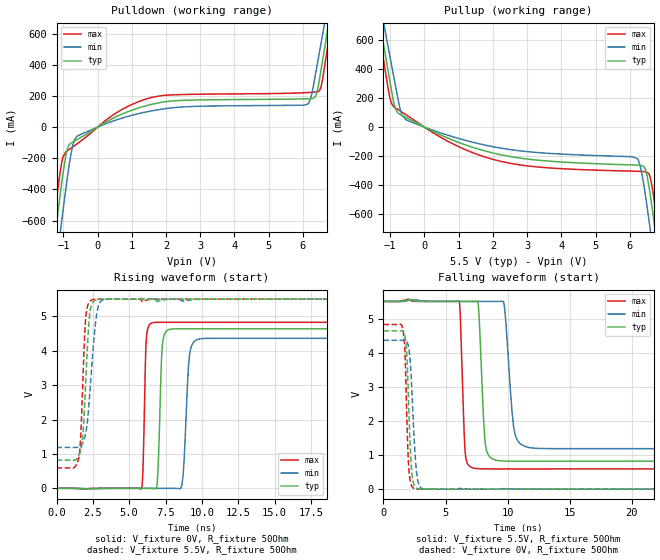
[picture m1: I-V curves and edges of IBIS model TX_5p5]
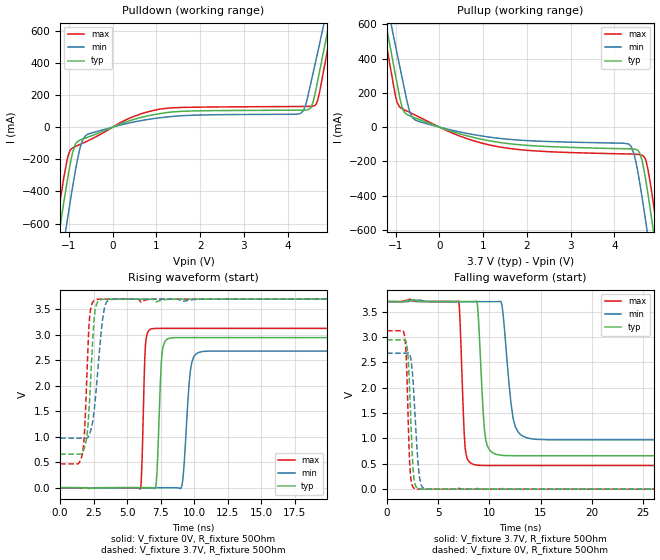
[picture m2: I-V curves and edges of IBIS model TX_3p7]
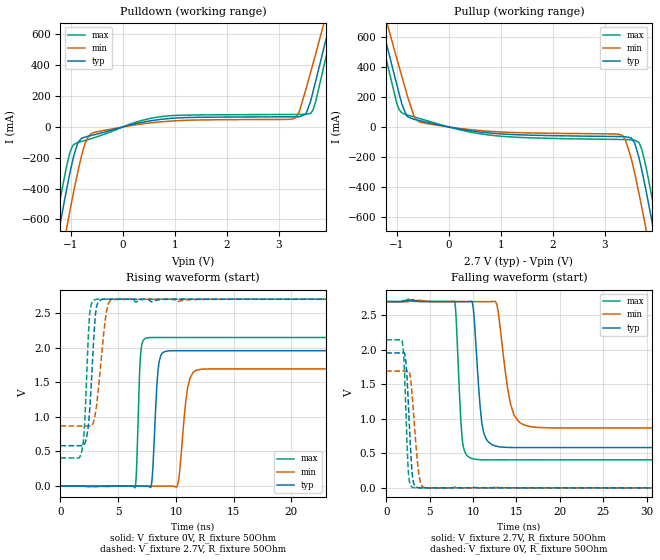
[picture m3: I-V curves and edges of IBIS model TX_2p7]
|Texas Instruments Incorporated
| Marketing part#   Digital Voltage Range   Package-type   #pins
| TDC1000QPWQ1   2.7V-5.5V   TSSOP   28
| TDC1000QPWRQ1   2.7V-5.5V   TSSOP   28
[IBIS Ver]   4.1
[File name]   tdc1000.ibs
[File Rev]   1.0
[Date]   09/30/2014
[Source]
| Texas Instruments Incorporated.
| 12500 TI Blvd
| Dallas, TX -75243
[Notes]   Revision History:
| Rev 1.0: 09/30/2014
| - Initial version of the model
| - Model generated from simulations in TISPICE
| - C_comp although listed in numerical order of value are
|   obtained from varying PVT conditions. For PVT conditions for
|   each specific value refer the buffer description under
|   respective [Model]. IBIS model user is responsible for using
|   appropriate C_comp to simulate for Signal Integrity.
| - Warnings regarding combined Non-monotonicity of various models have been
|   reviewd and considered minor and can be ignored.
| - Model names with a trailing _2p7 contains the model for
|   2.7V operation. Model names with a trailing _3p7 contains the model
|   for 3.7V operation. Model names with a trailing _5p5 contains the model
|   for 5.5V operation.
[Disclaimer]
| This model is designed as an aid for customers of Texas Instruments.
| TI and its licensors and suppliers make no warranties, either expressed
| or implied, with respect to this  model, including the warranties of
| merchantability or fitness for a particular purpose. The model is
| provided solely on an "as is" basis. The entire risk as to its quality
| and performance is with the customer.
[Copyright]
 (C) Copyright 2014 Texas Instruments Incorporated.All rights reserved.
|   Device
[Component]   TDC1000
[Manufacturer]   TI
[Package]   |TSSOP   28
|   typ   min   max
R_pkg   0.115   0.063   0.148
L_pkg   2.909nH   2.079nH   4.166nH
C_pkg   0.519pF   0.426pF   0.680pF
[Pin]  signal_name   model_name   R_pin   L_pin   C_pin
1   RX1   NC   0.1479   4.16158nH   0.6765pF
2   RX2   NC   0.1397   3.68744nH   0.64936pF
3   VCOM   NC   0.13246   3.07805nH   0.50984pF
4   LNA_OUT   NC   0.12659   2.75614nH   0.45467pF
5   PGA_IN   NC   0.10776   2.43486nH   0.45346pF
6   PGA_OUT   NC   0.09293   2.18856nH   0.43531pF
7   COMP_IN   NC   0.08627   2.07927nH   0.42641pF
8   RTD1   NC   0.08707   2.09237nH   0.42724pF
9   RTD2   NC   0.09713   2.25756nH   0.43859pF
10   RREF   NC   0.11109   2.49003nH   0.4531pF
11   CHSEL   CLKIN   0.12582   2.74301nH   0.44963pF
12   ERRB   ERRB   0.13589   3.13398nH   0.5143pF
13   START   START   0.1415   3.71632nH   0.65514pF
14   STOP   START   0.14784   4.16018nH   0.67999pF
15   EN   CLKIN   0.1476   4.15828nH   0.67882pF
16   TRIGGER   CLKIN   0.1406   3.70502nH   0.65246pF
17   RESET   CLKIN   0.13387   3.10558nH   0.51163pF
18   SCLK   CLKIN   0.12696   2.76761nH   0.45522pF
19   CSB   CLKIN   0.10764   2.43933nH   0.45435pF
20   SDI   CLKIN   0.09259   2.19086nH   0.43561pF
21   SDO   SDO   0.08627   2.08818nH   0.42716pF
22   VIO   POWER   0.08779   2.11267nH   0.42657pF
23   VDD   POWER   0.09343   2.20456nH   0.436pF
24   VDD   POWER   0.06304   2.24215nH   0.49177pF
25   CLKIN   CLKIN   0.12549   2.74304nH   0.45791pF
26   GND   GND   0.07953   2.81241nH   0.56155pF
27   TX2   TX   0.14161   3.72304nH   0.65349pF
28   TX1   TX   0.14806   4.16648nH   0.67973pF
|   Model Selectors
[Model Selector]  CLKIN
CLKIN_3p7   input buffer at 3.7V operation.
CLKIN_2p7   input buffer at 2.7V operation.
CLKIN_5p5   input buffer at 5.5V operation.
[Model Selector]  SDO
SDO_3p7   SDO buffer at 3.7V operation.
SDO_2p7   SDO buffer at 2.7V operation.
SDO_5p5   SDO buffer at 5.5V operation.
[Model Selector]  ERRB
ERRB_3p7   ERRB buffer at 3.7V operation.
ERRB_2p7   ERRB buffer at 2.7V operation.
ERRB_5p5   ERRB buffer at 5.5V operation.
[Model Selector]  START
START_3p7   START buffer at 3.7V operation.
START_2p7   START buffer at 2.7V operation.
START_5p5   START buffer at 5.5V operation.
[Model Selector]  TX
TX_3p7   TX buffer at 3.7V operation.
TX_2p7   TX buffer at 2.7V operation.
TX_5p5   TX buffer at 5.5V operation.
| Models and submodels in the file (15): TX_5p5 (Output), TX_3p7 (Output), TX_2p7 (Output), START_5p5 (Output), START_3p7 (Output), START_2p7 (Output), SDO_5p5 (I/O), SDO_3p7 (I/O), SDO_2p7 (I/O), ERRB_5p5 (Open_drain), ERRB_3p7 (Open_drain), ERRB_2p7 (Open_drain), CLKIN_5p5 (Input), CLKIN_3p7 (Input), CLKIN_2p7 (Input)
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|   Model
[Model]   TX_5p5
Model_type   Output
Polarity   Non-Inverting
Vmeas = 2.25
Vref = 0
Cref = 1pF
Rref = 100000
|   typ   min   max
C_comp   1.444pF   1.410pF   1.465pF
[Voltage Range]   5.5   5.499   5.501
[Temperature Range]   27   125   -40
[Pullup Reference]   5.5   5.499   5.501
[Pulldown Reference]   0   -0   -0
[Power Clamp Reference]   5.5   5.499   5.501
[GND Clamp Reference]   0   0   0
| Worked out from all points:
|   slope of the pulldown table from 0 to 0.825 V, typ, clamps not added: 8.8 ohm
|   slope of the pullup table from 0 to 0.825 V, typ, clamps not added: 9.26 ohm
|   falling waveform, V_fixture 5.5V, R_fixture 50Ohm: 20-80 % time 343ps typ, 512ps min, 269ps max; typ from 5.5 V to 0.82 V
|   rising waveform, V_fixture 0V, R_fixture 50Ohm: 20-80 % time 201ps typ, 289ps min, 154ps max; typ from 0 V to 4.64 V
|   rising waveform, V_fixture 5.5V, R_fixture 50Ohm: 20-80 % time 342ps typ, 487ps min, 273ps max; typ from 0.819 V to 5.5 V
|   falling waveform, V_fixture 0V, R_fixture 50Ohm: 20-80 % time 289ps typ, 373ps min, 242ps max; typ from 4.64 V to 0 V
[Pulldown]
|   Voltage   I(typ)   I(min)   I(max)
-5.5V     -8.576A    -8.65A     -8.542A
-1.359V   -911.3mA   -1.16A     -751.2mA
-1.194V   -608mA     -862.5mA   -451.1mA
-1.078V   -405.1mA   -654.4mA   -264.9mA
-731.5mV  -96.28mA   -123mA     -128mA
-451mV    -61.4mA    -42.19mA   -83.13mA
1.628V    148.9mA    106.4mA    193.1mA
6.133V    182.2mA    146.9mA    221.8mA
6.495V    320.8mA    496.1mA    238.5mA
6.726V    633.4mA    783.1mA    523.8mA
6.875V    836.9mA    971.3mA    741mA
11V       6.743A     6.524A     6.958A
[Pullup]
|   Voltage   I(typ)   I(min)   I(max)
-5.5V     6.748A     6.532A     6.959A
-1.359V   794.9mA    928.5mA    700.8mA
-1.144V   499mA      654.7mA    385.6mA
-962.5mV  251.7mA    427.6mA    161.7mA
-649mV    79.98mA    80.32mA    102.1mA
473mV     -53.82mA   -39.58mA   -69.9mA
6.215V    -261.2mA   -215.3mA   -303.8mA
6.446V    -285.5mA   -452.7mA   -307.9mA
6.595V    -459.4mA   -700.9mA   -343.6mA
6.726V    -682.6mA   -937mA     -526.3mA
6.875V    -953mA     -1.205A    -790mA
11V       -8.585A    -8.662A    -8.547A
[Ramp]
R_load = 50
|   typ   min   max
dV/dt_r   2.78207/2.01238e-10   2.61637/2.89224e-10   2.89484/1.53585e-10
dV/dt_f   2.80772/3.43261e-10   2.58647/5.11565e-10   2.94405/2.68906e-10
[Falling Waveform]
V_fixture = 5.5V
V_fixture_min = 5.499V
V_fixture_max = 5.501V
R_fixture = 50Ohm
C_fixture = 0F
|   Time   V(typ)   V(min)   V(max)
0s        5.5V       5.499V     5.501V
6.105ns   5.501V     5.5V       5.51V
6.567ns   5.5V       5.5V       1.156V
7.282ns   5.5V       5.5V       616.1mV
7.643ns   5.397V     5.499V     600.4mV
8.212ns   1.305V     5.499V     595mV
9.098ns   846.1mV    5.499V     594mV
10.49ns   819.5mV    1.807V     594mV
11.43ns   818.9mV    1.249V     594mV
50ns      820.5mV    1.188V     594.3mV
[Rising Waveform]
V_fixture = 0V
V_fixture_min = 0V
V_fixture_max = 0V
R_fixture = 50Ohm
C_fixture = 0F
|   Time   V(typ)   V(min)   V(max)
0s        7.238uV    3.34uV     -5.404uV
5.826ns   63.71uV    -314.4uV   -24.46mV
6.165ns   75.83uV    -304uV     4.245V
6.626ns   -3.01mV    -289.9uV   4.816V
7.285ns   4.173V     -269.8uV   4.825V
7.808ns   4.623V     -253.8uV   4.825V
8.629ns   4.637V     84.19mV    4.825V
9.158ns   4.637V     3.9V       4.825V
9.838ns   4.637V     4.342V     4.825V
50ns      4.637V     4.361V     4.825V
[Rising Waveform]
V_fixture = 5.5V
V_fixture_min = 5.499V
V_fixture_max = 5.501V
R_fixture = 50Ohm
C_fixture = 0F
|   Time   V(typ)   V(min)   V(max)
0s        818.9mV    1.187V     594.3mV
1.302ns   820.3mV    1.189V     643.1mV
1.677ns   1.14V      1.219V     1.622V
1.849ns   1.772V     1.365V     3.53V
2.022ns   3.215V     1.629V     5.019V
2.234ns   4.86V      2.452V     5.4V
2.476ns   5.394V     3.832V     5.484V
2.912ns   5.495V     5.358V     5.499V
3.384ns   5.498V     5.493V     5.499V
50ns      5.5V       5.499V     5.501V
[Falling Waveform]
|Gnd
V_fixture = 0V
V_fixture_min = 0V
V_fixture_max = 0V
R_fixture = 50Ohm
C_fixture = 0F
|   Time   V(typ)   V(min)   V(max)
0s        4.637V     4.361V     4.825V
1.452ns   4.639V     4.363V     4.817V
1.735ns   4.476V     4.364V     4.002V
1.849ns   4.156V     4.35V      2.611V
2.022ns   2.619V     4.168V     737.4mV
2.234ns   722.5mV    3.315V     135.5mV
2.476ns   111mV      1.475V     17.85mV
2.761ns   13.14mV    250.3mV    3.519mV
3.275ns   1.59mV     6.61mV     12.82uV
50ns      -7.24uV    -3.313uV   -5.406uV
|   Model
[Model]   TX_3p7
Model_type   Output
Polarity   Non-Inverting
Vmeas = 1.85
Vref = 0
Cref = 1pF
Rref = 100000
|   typ   min   max
C_comp   1.444pF   1.410pF   1.465pF
[Voltage Range]   3.7   3.699   3.701
[Temperature Range]   27   125   -40
[Pullup Reference]   3.7   3.699   3.701
[Pulldown Reference]   -0   0   0
[Power Clamp Reference]   3.7   3.699   3.701
[GND Clamp Reference]   0   0   0
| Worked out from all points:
|   slope of the pulldown table from 0 to 0.555 V, typ, clamps not added: 10.4 ohm
|   slope of the pullup table from 0 to 0.555 V, typ, clamps not added: 12.2 ohm
|   falling waveform, V_fixture 3.7V, R_fixture 50Ohm: 20-80 % time 481ps typ, 760ps min, 354ps max; typ from 3.7 V to 0.659 V
|   rising waveform, V_fixture 0V, R_fixture 50Ohm: 20-80 % time 254ps typ, 392ps min, 190ps max; typ from 0 V to 2.94 V
|   rising waveform, V_fixture 3.7V, R_fixture 50Ohm: 20-80 % time 386ps typ, 565ps min, 307ps max; typ from 0.659 V to 3.7 V
|   falling waveform, V_fixture 0V, R_fixture 50Ohm: 20-80 % time 367ps typ, 487ps min, 293ps max; typ from 2.94 V to 0 V
[Pulldown]
|   Voltage   I(typ)   I(min)   I(max)
-3.7V     -5.24A     -5.387A    -5.152A
-1.236V   -682.9mA   -937.3mA   -522.6mA
-1.103V   -444.1mA   -697.1mA   -293.6mA
-980.5mV  -244.5mA   -481.5mA   -149mA
-847.3mV  -103.8mA   -264.5mA   -119.9mA
-580.9mV  -63.79mA   -45.98mA   -86.98mA
1.073V    83.95mA    58.06mA    111.5mA
4.281V    105.7mA    83.79mA    128.6mA
4.525V    118.4mA    264.4mA    129.3mA
4.669V    260mA      440.4mA    152.1mA
5.08V     819.2mA    955.4mA    721.7mA
7.4V      4.118A     4.051A     4.198A
[Pullup]
|   Voltage   I(typ)   I(min)   I(max)
-3.7V     4.128A     4.059A     4.21A
-1.247V   632mA      778mA      527.3mA
-969.4mV  253.1mA    429.4mA    145.1mA
-691.9mV  67.26mA    99.5mA     87.25mA
-492.1mV  47.45mA    35.02mA    62.44mA
1.406V    -90.69mA   -66.52mA   -117.2mA
4.325V    -126.6mA   -99.07mA   -156.6mA
4.581V    -151.8mA   -326.6mA   -160.8mA
4.758V    -374.5mA   -623.8mA   -235.9mA
4.847V    -526.3mA   -782.8mA   -369.1mA
4.969V    -747mA     -1.003A    -583.6mA
7.4V      -5.242A    -5.392A    -5.151A
[Ramp]
R_load = 50
|   typ   min   max
dV/dt_r   1.76687/2.53519e-10   1.60881/3.92443e-10   1.87534/1.89844e-10
dV/dt_f   1.82442/4.8142e-10   1.63586/7.59731e-10   1.94062/3.53705e-10
[Falling Waveform]
V_fixture = 3.7V
V_fixture_min = 3.699V
V_fixture_max = 3.701V
R_fixture = 50Ohm
C_fixture = 0F
|   Time   V(typ)   V(min)   V(max)
0s        3.7V       3.699V     3.701V
7.009ns   3.7V       3.699V     3.706V
7.63ns    3.7V       3.699V     823mV
8.487ns   3.7V       3.699V     485.6mV
8.865ns   3.579V     3.699V     473.6mV
9.656ns   966.3mV    3.699V     466.8mV
10.74ns   682.9mV    3.7V       466.3mV
12.32ns   660mV      1.4V       466.3mV
13.6ns    659.3mV    1.016V     466.3mV
50ns      659.3mV    972.6mV    466.6mV
[Rising Waveform]
V_fixture = 0V
V_fixture_min = 0V
V_fixture_max = 0V
R_fixture = 50Ohm
C_fixture = 0F
|   Time   V(typ)   V(min)   V(max)
0s        66.29nV    655.2nV    5.051uV
6.007ns   156.6uV    -100.2uV   -14.37mV
6.369ns   195uV      -65.25uV   2.794V
6.808ns   -388.4uV   -22.71uV   3.116V
7.606ns   2.631V     54.46uV    3.126V
8.117ns   2.93V      103.9uV    3.126V
9.095ns   2.945V     40.51mV    3.126V
9.712ns   2.945V     2.273V     3.126V
10.54ns   2.945V     2.668V     3.126V
50ns      2.945V     2.681V     3.126V
[Rising Waveform]
V_fixture = 3.7V
V_fixture_min = 3.699V
V_fixture_max = 3.701V
R_fixture = 50Ohm
C_fixture = 0F
|   Time   V(typ)   V(min)   V(max)
0s        658.8mV    972.6mV    466.6mV
1.499ns   658.7mV    971.8mV    528.4mV
1.731ns   726.2mV    971.7mV    785.4mV
1.899ns   866.9mV    971.6mV    1.544V
2.212ns   1.792V     1.066V     3.39V
2.541ns   3.329V     1.519V     3.674V
2.742ns   3.613V     2.086V     3.695V
3.314ns   3.698V     3.542V     3.7V
3.757ns   3.699V     3.691V     3.7V
50ns      3.7V       3.699V     3.701V
[Falling Waveform]
|Gnd
V_fixture = 0V
V_fixture_min = 0V
V_fixture_max = 0V
R_fixture = 50Ohm
C_fixture = 0F
|   Time   V(typ)   V(min)   V(max)
0s        2.945V     2.681V     3.126V
1.574ns   2.945V     2.681V     3.125V
1.899ns   2.876V     2.682V     2.498V
2.09ns    2.507V     2.685V     1.22V
2.275ns   1.639V     2.622V     312.1mV
2.541ns   416.5mV    2.131V     39.7mV
2.742ns   98mV       1.444V     7.987mV
3.162ns   5.161mV    247.8mV    797.2uV
3.757ns   642.2uV    5.884mV    658.4uV
50ns      -69.49nV   663.3nV    5.052uV
|   Model
[Model]   TX_2p7
Model_type   Output
Polarity   Non-Inverting
Vmeas = 1.35
Vref = 0
Cref = 1pF
Rref = 100000
|   typ   min   max
C_comp   1.444pF   1.410pF   1.465pF
[Voltage Range]   2.7   2.699   2.701
[Temperature Range]   27   125   -40
[Pullup Reference]   2.7   2.699   2.701
[Pulldown Reference]   0   -0   0
[Power Clamp Reference]   2.7   2.699   2.701
[GND Clamp Reference]   0   0   0
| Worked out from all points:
|   slope of the pulldown table from 0 to 0.405 V, typ, clamps not added: 12.6 ohm
|   slope of the pullup table from 0 to 0.405 V, typ, clamps not added: 16.4 ohm
|   falling waveform, V_fixture 2.7V, R_fixture 50Ohm: 20-80 % time 731ps typ, 1.17ns min, 523ps max; typ from 2.7 V to 0.584 V
|   rising waveform, V_fixture 0V, R_fixture 50Ohm: 20-80 % time 356ps typ, 570ps min, 249ps max; typ from 0 V to 1.96 V
|   rising waveform, V_fixture 2.7V, R_fixture 50Ohm: 20-80 % time 450ps typ, 661ps min, 359ps max; typ from 0.584 V to 2.7 V
|   falling waveform, V_fixture 0V, R_fixture 50Ohm: 20-80 % time 479ps typ, 648ps min, 373ps max; typ from 1.96 V to 0 V
[Pulldown]
|   Voltage   I(typ)   I(min)   I(max)
-2.7V     -3.388A    -3.578A    -3.269A
-1.323V   -842.6mA   -1.094A    -680.9mA
-1.234V   -678.1mA   -932.9mA   -516.8mA
-1.08V    -402.7mA   -655.4mA   -252.8mA
-861.3mV  -100.8mA   -283.6mA   -101.4mA
-666.9mV  -60.22mA   -62.7mA    -81.67mA
126.9mV   11.86mA    7.573mA    17.23mA
3.27V     65.77mA    52.56mA    80.85mA
3.61V     167.3mA    355.2mA    88.61mA
3.715V    308.5mA    484.6mA    177.1mA
4.128V    873.5mA    1.006A     779.9mA
5.4V      2.672A     2.69A      2.678A
[Pullup]
|   Voltage   I(typ)   I(min)   I(max)
-2.7V     2.681A     2.696A     2.69A
-1.388V   820.4mA    953.4mA    727.5mA
-990.9mV  276.2mA    451.3mA    153mA
-788.4mV  68.16mA    202.3mA    79.31mA
-513mV    38.78mA    29.03mA    51.69mA
872.1mV   -43.15mA   -31.21mA   -57.72mA
3.229V    -64.04mA   -47.44mA   -83.46mA
3.505V    -73.01mA   -202.8mA   -86.27mA
3.667V    -217.5mA   -458.3mA   -110.1mA
3.804V    -443.7mA   -701.2mA   -285.8mA
4.023V    -841.8mA   -1.096A    -677.6mA
5.4V      -3.387A    -3.58A     -3.266A
[Ramp]
R_load = 50
|   typ   min   max
dV/dt_r   1.17346/3.55763e-10   1.01572/5.69708e-10   1.288/2.48756e-10
dV/dt_f   1.26984/7.31513e-10   1.09827/1.17127e-09   1.37641/5.22576e-10
[Falling Waveform]
V_fixture = 2.7V
V_fixture_min = 2.699V
V_fixture_max = 2.701V
R_fixture = 50Ohm
C_fixture = 0F
|   Time   V(typ)   V(min)   V(max)
0s        2.7V       2.699V     2.701V
7.837ns   2.7V       2.699V     2.708V
8.751ns   2.7V       2.699V     711.7mV
9.754ns   2.704V     2.699V     431mV
11.03ns   932.7mV    2.699V     407.4mV
12.19ns   626.2mV    2.701V     405.9mV
12.91ns   598.5mV    2.553V     406.7mV
14.33ns   585mV      1.214V     405.7mV
16.1ns    584.2mV    903.3mV    406.9mV
50ns      583.6mV    868.5mV    407mV
[Rising Waveform]
V_fixture = 0V
V_fixture_min = 0V
V_fixture_max = 0V
R_fixture = 50Ohm
C_fixture = 0F
|   Time   V(typ)   V(min)   V(max)
0s        -5.1uV     2.2uV      -928.5nV
6.457ns   35.4uV     -270.9uV   -26.49mV
6.913ns   150.3uV    -199.1uV   1.844V
7.434ns   183.7uV    -117uV     2.139V
7.866ns   747.3uV    -48.99uV   2.146V
9.062ns   1.945V     139.5uV    2.147V
10.15ns   1.956V     11.57mV    2.147V
11.02ns   1.956V     1.418V     2.147V
11.94ns   1.956V     1.681V     2.147V
50ns      1.956V     1.693V     2.147V
[Rising Waveform]
V_fixture = 2.7V
V_fixture_min = 2.699V
V_fixture_max = 2.701V
R_fixture = 50Ohm
C_fixture = 0F
|   Time   V(typ)   V(min)   V(max)
0s        583.8mV    868.3mV    406mV
1.866ns   582.1mV    866.7mV    519.2mV
2.113ns   616.3mV    866.5mV    960.3mV
2.502ns   1.037V     866.2mV    2.437V
2.661ns   1.455V     866mV      2.622V
3.013ns   2.437V     1.039V     2.695V
3.249ns   2.654V     1.345V     2.7V
3.963ns   2.699V     2.506V     2.7V
4.506ns   2.7V       2.693V     2.7V
50ns      2.7V       2.699V     2.701V
[Falling Waveform]
|Gnd
V_fixture = 0V
V_fixture_min = 0V
V_fixture_max = 0V
R_fixture = 50Ohm
C_fixture = 0F
|   Time   V(typ)   V(min)   V(max)
0s        1.956V     1.693V     2.147V
1.866ns   1.956V     1.693V     2.106V
2.026ns   1.96V      1.693V     1.898V
2.222ns   1.874V     1.693V     1.297V
2.407ns   1.574V     1.694V     614.5mV
2.576ns   1.158V     1.697V     192.5mV
3.013ns   195.1mV    1.312V     8.514mV
3.768ns   2.219mV    189.6mV    144.4uV
4.331ns   800.9uV    8.635mV    3.809uV
50ns      5.13uV     -2.175uV   -1.539uV
